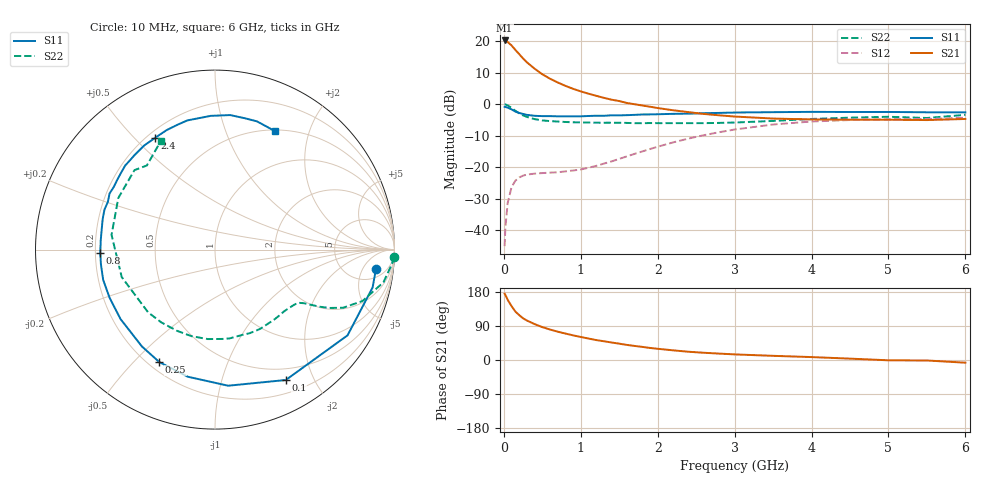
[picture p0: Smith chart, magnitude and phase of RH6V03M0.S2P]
! SIEMENS Small Signal Semiconductors
! BFR106
! Si NPN RF Bipolar Junction Transistor in SOT23
! VCE = 6 V  IC = 3 mA
! Common Emitter S-Parameters:  August  1996
# GHz  S  MA  R  50
!  f  S11  S21  S12  S22
! GHz  MAG  ANG  MAG  ANG  MAG  ANG  MAG  ANG
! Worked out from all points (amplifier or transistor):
!   36 points, 10 MHz to 6 GHz, reference 50 ohm
!   highest |S21| = 20.2 dB at 10 MHz (marker M1)
!   |S21| within 3 dB of that: start of sweep to 149.9 MHz
!   unconditionally stable (mu >= 1): 720.5 MHz to 1.825 GHz; 4.429 GHz to end of sweep
!   at 250 MHz: K = 0.38, MSG = 18.6 dB, |S12| = -22.7 dB
!   at 1.4 GHz: K = 1.17, MAG = 7.3 dB, |S12| = -18.2 dB
!   at 6 GHz: K = 1.02, MAG = -1.0 dB, |S12| = -4.3 dB
!   S11 on the Smith chart (normalised r, x): 10 MHz: 8, -10; 100 MHz: 0.35, -1.62; 250 MHz: 0.24, -0.59; 800 MHz: 0.22, -0.01; 2.4 GHz: 0.23, +0.58; 6 GHz: 0.51, +1.50
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0.01  0.9033 -6.7  10.22 175.0  0.0056 88.1  0.9965 -2.3
0.02  0.9032 -13.5  10.18 171.6  0.0111 83.8  0.9896 -4.6
0.05  0.8795 -32.9  9.659 158.8  0.0272 73.5  0.956 -11.0
0.1  0.8267 -61.5  8.528 142.2  0.0482 58.7  0.8704 -19.2
0.15  0.7619 -84.5  7.235 127.9  0.0612 48.6  0.7842 -24.4
0.2  0.7243 -102.1  6.204 118.4  0.0688 42.3  0.7162 -27.0
0.25  0.699 -116.4  5.294 110.0  0.0735 37.7  0.6623 -28.7
0.3  0.6761 -127.0  4.597 104.2  0.0765 35.6  0.6277 -29.6
0.4  0.6533 -143.7  3.647 94.7  0.0791 33.0  0.5782 -31.1
0.5  0.6457 -155.5  2.976 86.8  0.0807 33.1  0.5516 -32.5
0.6  0.6454 -164.9  2.531 80.4  0.0821 34.7  0.5387 -34.6
0.8  0.6394 -178.5  1.95 69.8  0.0858 40.9  0.5216 -39.6
1.1  0.6488 164.7  1.465 56.6  0.098 53.5  0.5111 -49.0
1.6  0.669 144.6  1.043 39.8  0.1486 67.2  0.504 -67.7
2.2  0.7015 124.2  0.8 25.5  0.2474 67.0  0.5001 -94.6
2.4  0.7066 118.1  0.747 21.8  0.2847 64.4  0.4998 -105.2
3.5  0.7456 91.8  0.591 11.0  0.4756 41.9  0.5417 -163.6
4  0.7542 83.6  0.572 7.7  0.5305 30.4  0.5822 171.9
4.5  0.7505 77.3  0.567 3.6  0.5602 20.1  0.6106 151.9
5  0.7518 71.9  0.566 -0.8  0.5759 11.4  0.6304 135.4
5.5  0.7425 66.6  0.559 -1.3  0.5803 7.1  0.6031 129.0
6  0.7397 63.3  0.582 -7.1  0.6089 -1.2  0.6763 116.5
